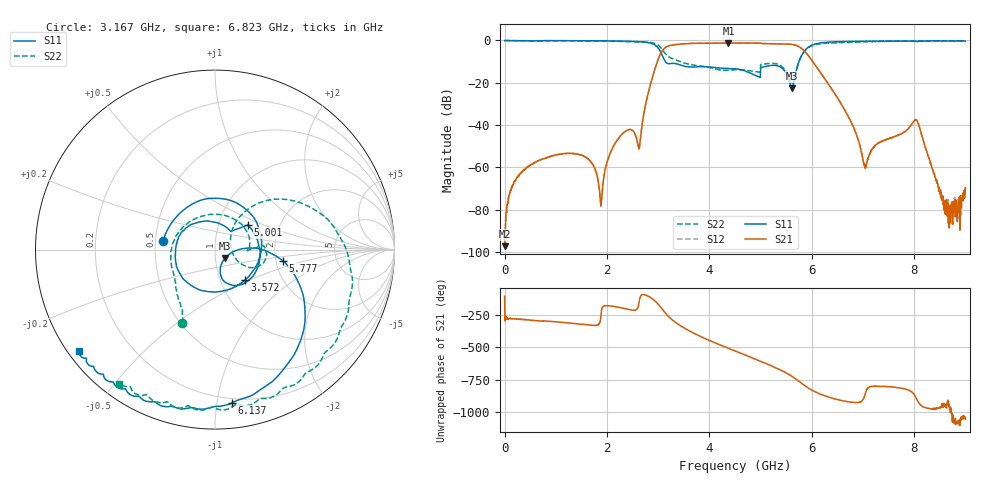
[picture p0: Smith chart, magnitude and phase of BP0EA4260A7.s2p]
!Agilent Technologies,E8358A,US40260310,A.06.04.32
!Agilent E8358A: A.06.04.32
!Date: Friday, November 22, 2019 00:22:04
!Correction: S11(Full 2 Port(1,2)) S21(Full 2 Port(1,2)) S12(Full 2 Port(1,2)) S22(Full 2 Port(1,2))
!S2P File: Measurements: S11, S21, S12, S22:
# Hz S  dB  R 50
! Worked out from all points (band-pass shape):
!   1601 points, 300 kHz to 9 GHz, reference 50 ohm
!   highest |S21| = -1.18 dB at 4.371 GHz (marker M1); lowest = -97.2 dB at 300 kHz (marker M2)
!   |S21| within 3 dB of the highest: 3.103 GHz to 5.817 GHz (2.714 GHz wide, 60.9 % of centre)
!   lowest |S11| = -22.6 dB at 5.614 GHz (marker M3), VSWR 1.16, Z = 55.8 - j5.22 ohm
!   |S11| at or under -10 dB: 3.141 GHz to 5.75 GHz (2.609 GHz wide, 58.7 % of centre)
!   |S22| runs from -21.0 to 0.0 dB; largest |S21 - S12| = 0.01
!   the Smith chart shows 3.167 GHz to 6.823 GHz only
!   S11 on the Smith chart (normalised r, x): 3.167 GHz: 0.55, +0.06; 3.572 GHz: 1.31, -0.47; 5.001 GHz: 1.38, +0.40; 5.777 GHz: 2.18, -0.32; 6.137 GHz: 0.17, -1.10; 6.823 GHz: 0.03, -0.33
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300000  -0.07 -180.0  -97.17 -106.1  -91.03 -104.4  -0.02 -179.9
4.50285e8  -0.15 169.5  -59.81 71.6  -59.75 71.4  -0.18 160.6
1.502125e9  -0.16 143.3  -54.25 37.6  -54.15 37.5  -0.25 111.6
1.884612e9  -0.20 128.3  -76.84 112.0  -77.43 116.0  -0.31 86.6
2.222101e9  -0.33 109.6  -46.35 169.1  -46.30 168.8  -0.48 55.9
2.627087e9  -0.61 70.6  -51.16 -151.4  -51.11 -151.1  -0.68 -0.3
3.00395e9  -3.69 -44.6  -8.65 -169.6  -8.58 -169.6  -2.29 -84.6
3.167069e9  -10.69 170.1  -2.95 111.7  -2.90 111.5  -6.97 -114.2
3.572056e9  -12.45 -44.9  -1.51 -5.4  -1.45 -5.6  -11.13 -143.2
4.370779e9  -13.23 173.9  -1.18 -147.0  -1.13 -147.2  -14.05 72.8
4.50015e9  -13.37 160.7  -1.19 -167.2  -1.14 -167.5  -13.82 45.4
5.000758e9  -12.82 36.8  -1.42 113.1  -1.38 113.0  -11.42 5.1
5.613863e9  -22.65 -39.1  -1.88 -3.4  -1.83 -3.6  -20.96 10.9
5.776982e9  -8.34 -9.3  -3.36 -49.8  -3.35 -49.8  -8.36 44.7
6.001975e9  -2.25 -60.9  -9.44 -109.2  -9.34 -109.5  -2.48 -5.2
6.13697e9  -1.32 -83.7  -14.07 -134.8  -13.98 -135.5  -1.67 -31.2
6.823198e9  -0.50 -143.4  -41.50 155.5  -41.45 156.1  -0.72 -125.4
7.042565e9  -0.43 -153.2  -60.15 -140.2  -60.53 -138.1  -0.73 -146.2
7.5038e9  -0.29 -170.0  -46.42 -82.8  -46.29 -83.7  -0.45 -173.8
8.038157e9  -0.37 175.4  -37.35 -169.6  -37.45 -169.3  -0.37 170.2
8.611888e9  -0.23 164.5  -82.19 138.9  -77.06 125.1  -0.23 158.6
9e9  -0.29 157.2  -69.63 26.1  -70.37 39.6  -0.20 152.4
